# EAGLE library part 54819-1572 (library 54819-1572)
USB Connectors USB Ser Mini-B Rec H sgAssy 5CktEmbsTpPkg Source: Datasheet
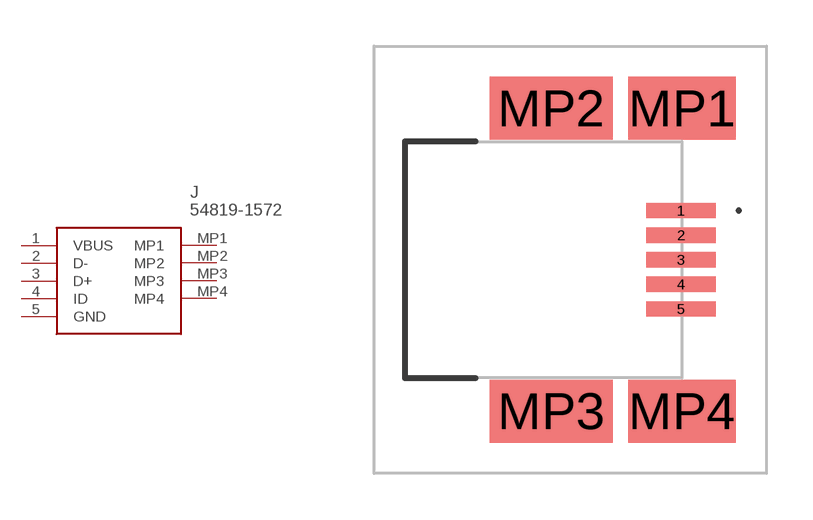
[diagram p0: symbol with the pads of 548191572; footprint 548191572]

Designator prefix J

## 54819-1572 (Description: USB Connectors USB Ser Mini-B Rec H sgAssy 5CktEmbsTpPkg; Height: 4.15mm; Manufacturer_Name: Molex; Manufacturer_Part_Number: 54819-1572; Mouser_Part_Number: 538-54819-1572; Mouser_Price-Stock: https://www.mouser.co.uk/ProductDetail/Molex/54819-1572?qs=S7M4C5ZllW4l%2FiJ3ZkbS7A%3D%3D)  [548191572]
1  VBUS
2  D-
3  D+
4  ID
5  GND
MP1  MP1
MP2  MP2
MP3  MP3
MP4  MP4

## Footprint 548191572 (pad centres in mm)
54819-1572-2
smd 2.25 x 0.5: 1 4.475,1.6; 2 4.475,0.8; 3 4.475,0; 4 4.475,-0.8; 5 4.475,-1.6
smd 3.5 x 2.05: MP1 4.5,4.925; MP4 4.5,-4.925
smd 4 x 2.05: MP2 0.25,4.925; MP3 0.25,-4.925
